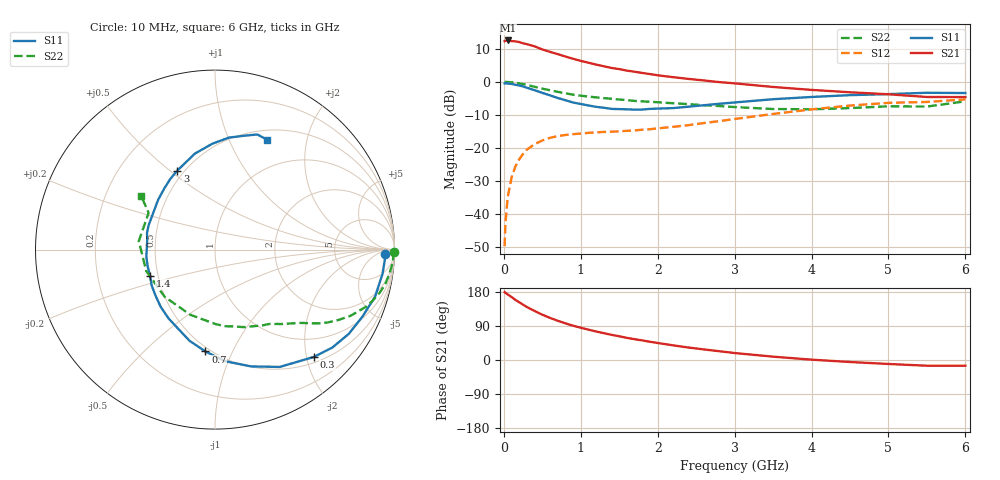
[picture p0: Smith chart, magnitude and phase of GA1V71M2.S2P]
! Infineon Technologies  Discrete & RF Semiconductors
! BF775
! Si NPN RF Bipolar Junction Transistor in SOT23
! VCE = 1.75 V  IC = 1.2 mA
! Common Emitter S-Parameters:  May  1996
# GHz  S  MA  R  50
!  f  S11  S21  S12  S22
! GHz  MAG  ANG  MAG  ANG  MAG  ANG  MAG  ANG
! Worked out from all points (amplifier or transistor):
!   36 points, 10 MHz to 6 GHz, reference 50 ohm
!   highest |S21| = 12.5 dB at 50 MHz (marker M1)
!   |S21| within 3 dB of that: start of sweep to 538.8 MHz
!   unconditionally stable (mu >= 1): 1.332 GHz to end of sweep
!   at 250 MHz: K = 0.23, MSG = 16.7 dB, |S12| = -21.8 dB
!   at 1.4 GHz: K = 1.05, MAG = 8.3 dB, |S12| = -15.1 dB
!   at 6 GHz: K = 1.05, MAG = -1.1 dB, |S12| = -5.3 dB
!   S11 on the Smith chart (normalised r, x): 10 MHz: 29, -14; 300 MHz: 0.61, -2.14; 700 MHz: 0.47, -0.79; 1.4 GHz: 0.45, -0.16; 3 GHz: 0.46, +0.53; 6 GHz: 0.62, +1.40
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0.01  0.9454 -1.6  4.111 179.1  0.0033 87.8  0.9987 -0.7
0.02  0.9483 -3.2  4.174 177.1  0.0071 83.9  0.9942 -1.6
0.05  0.9431 -8.3  4.21 173.1  0.0181 85.5  0.9935 -3.9
0.1  0.9295 -16.4  4.118 166.4  0.0358 80.4  0.9819 -7.7
0.15  0.902 -24.6  4.081 158.7  0.0526 74.8  0.9677 -11.5
0.2  0.8809 -32.2  3.982 152.3  0.0675 70.4  0.9469 -14.9
0.3  0.8135 -47.3  3.7 139.8  0.0946 62.1  0.8975 -20.9
0.4  0.7467 -61.1  3.434 129.5  0.1147 54.7  0.8408 -26.0
0.5  0.6813 -72.8  3.08 119.5  0.13 49.2  0.7876 -30.0
0.6  0.6248 -84.7  2.83 111.2  0.1427 44.6  0.746 -33.0
0.7  0.5698 -95.4  2.622 103.6  0.1514 41.2  0.7064 -35.6
0.9  0.4869 -114.8  2.228 90.5  0.1621 36.2  0.6398 -39.7
1.1  0.4394 -133.5  1.941 80.1  0.1696 33.5  0.5989 -43.3
1.4  0.39 -158.1  1.619 66.4  0.1765 31.7  0.5543 -48.5
1.7  0.3798 178.1  1.419 54.9  0.1843 33.6  0.5142 -53.6
2.2  0.4009 148.8  1.175 38.7  0.2088 36.6  0.4745 -64.4
3  0.4878 115.5  0.947 18.4  0.2745 38.1  0.4156 -89.4
3.5  0.5462 101.9  0.836 8.8  0.3271 35.2  0.3882 -110.8
4.5  0.6288 82.9  0.695 -5.3  0.4376 23.9  0.4011 -162.7
5  0.652 76.3  0.648 -10.5  0.4811 16.3  0.4272 173.6
5.5  0.6835 69.8  0.59 -15.1  0.4967 7.9  0.4227 151.0
6  0.6769 64.4  0.588 -15.0  0.5428 3.6  0.5073 144.1
